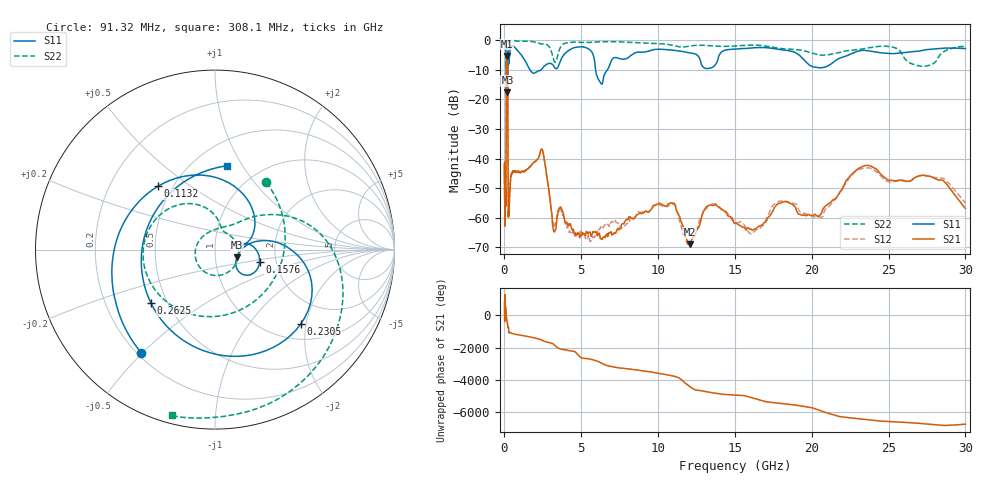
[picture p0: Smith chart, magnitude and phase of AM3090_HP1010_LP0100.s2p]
! Date/Time: Thu, Feb 28, 2019 2:04 PM
! Network Analyzer: Agilent Technologies E8364B Rev: A.07.50.67
! Sweep from 0.010 to 30.000 GHz, 1601 Points, Sweep Type: LOG
! Power Supply: 5.023 V, 0.002 A
# Hz S DB R 50
!freq MagS11 AngS11 MagS21 AngS21 MagS12 AngS12 MagS22 AngS22
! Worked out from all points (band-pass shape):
!   1601 points, 10 MHz to 30 GHz, reference 50 ohm
!   highest |S21| = -5.36 dB at 158.3 MHz (marker M1); lowest = -68.9 dB at 12.07 GHz (marker M2)
!   |S21| within 3 dB of the highest: 126.8 MHz to 200 MHz (73.23 MHz wide, 44.8 % of centre)
!   lowest |S11| = -17.7 dB at 190.6 MHz (marker M3), VSWR 1.30, Z = 63.8 - j5.52 ohm
!   |S11| at or under -10 dB: 123 MHz to 209.7 MHz (86.77 MHz wide, 52.2 % of centre); 1.65 GHz to 2.394 GHz (744.8 MHz wide, 36.8 % of centre); 5.927 GHz to 6.71 GHz (782.4 MHz wide, 12.4 % of centre)
!   |S22| runs from -20.0 to -0.1 dB; largest |S21 - S12| = 0.014
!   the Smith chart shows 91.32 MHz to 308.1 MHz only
!   S11 on the Smith chart (normalised r, x): 91.32 MHz: 0.22, -0.49; 113.2 MHz: 0.42, +0.38; 157.6 MHz: 1.64, -0.23; 230.5 MHz: 1.36, -1.87; 262.5 MHz: 0.41, -0.31; 308.1 MHz: 0.71, +0.86
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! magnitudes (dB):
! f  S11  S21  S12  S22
! 10 MHz  -0.2  -41.2  -48.8  -0.6
! 38.04 MHz  -0.5  -60.3  -59.8  -1.3
! 51.88 MHz  -0.8  -49.2  -45.9  -1.4
! 91.32 MHz  -3.0  -51.7  -53.5  -6.5
! 113.2 MHz  -6.5  -20.7  -20.7  -7.9
! 144.7 MHz  -14.0  -5.6  -5.5  -18.6
! 157.6 MHz  -11.8  -5.4  -5.3  -17.0
! 158.3 MHz  -11.8  -5.4  -5.3  -16.9
! 190.6 MHz  -17.7  -6.7  -6.7  -19.6
! 210.6 MHz  -9.6  -13.8  -13.8  -11.1
! 230.5 MHz  -4.0  -42.0  -41.7  -2.6
! 262.5 MHz  -6.6  -58.6  -58.1  -0.8
! 308.1 MHz  -6.5  -57.7  -54.9  -0.4
! 550.5 MHz  -2.0  -44.3  -44.7  -0.2
! 2.084 GHz  -10.8  -40.6  -40.4  -0.8
! 2.52 GHz  -9.2  -38.1  -38.0  -1.3
! 3.236 GHz  -9.1  -64.4  -62.0  -7.2
! 7.926 GHz  -6.3  -60.8  -62.0  -0.7
! 12.07 GHz  -4.3  -68.9  -69.3  -2.1
! 20 GHz  -8.9  -59.2  -59.4  -4.4
! 23.48 GHz  -3.5  -42.4  -43.2  -2.9
! 30 GHz  -2.9  -56.8  -55.0  -2.2
